FUNCTION_BLOCK FB81
TITLE =Get Target Velocity
//*****************************************************************************
//* maxon motor ag
//* R&D
//* all rights reserved
//*****************************************************************************
//* Summary:  Read target value of velocity
//*
//* Remarks:
//*
//* Created under: STEP7 REV5.2+SP1
//*****************************************************************************
//* History:
//* 19.05.2004 | INA   first release
//*
//*
//*****************************************************************************
//

AUTHOR:INA
FAMILY:ProVeloM
NAME:GetTarVe
VERSION:00.01


VAR_INPUT

Read : BOOL //A rising edge start the command

  NodeID : BYTE //Adress of the maxon device

END_VAR
VAR_OUTPUT
  Done : BOOL //Data valid flag is TRUE if data were available

  Err : BOOL //Error flag is TRUE if an Error has occured, see ErrNo for more details

  ErrNo : DINT //Contains detailed error information

  TargetVelocity : DINT //Target Velocity

END_VAR
VAR
  xEdgeMerker : BOOL //Edge Merker

  xEdgeFlag : BOOL //Edge Flag

  xStep : INT
END_VAR

BEGIN

NETWORK
TITLE = Activate the service function
//

// SDO Read "Get Target Velocity"

       U    #Read
       FP   #xEdgeFlag                   // recognize a positiv edge of the Read signal
       =    #xEdgeMerker                 // and set the xEdgeMerker for one cycle to true

       L    #xStep
       L    0
       ==I
       U    #xEdgeMerker
       SPB  nstp                         // iStep = 1 -> fnc1

       L    #xStep                       // jump list
       SPL  List
       SPA  rdef
       SPA  fnc1
       SPA  fncE
List  :SPA  rdef

rdef  :NOP  0
       R    #Done                        // reset Done
       R    #Err                         // reset Error
       L    0
       T    #xStep                       // iStep = 0
       SPA  end

fnc1  :NOP  0
       CALL FC1
         NodeID:=#NodeID
         Index:=DW#16#000060FF
         SubIndex:=DW#16#00000000
         RET_VAL:=#Done
         Err:=#Err
         ErrNo:=#ErrNo

       L    DB219.DBD10
       T    #TargetVelocity

fncE  :NOP  0
       L    0
       T    #xStep
       SPA  end

nstp  :NOP  0
       L    #xStep
       INC            1
       T    #xStep

end   :NOP  0
END_FUNCTION_BLOCK
